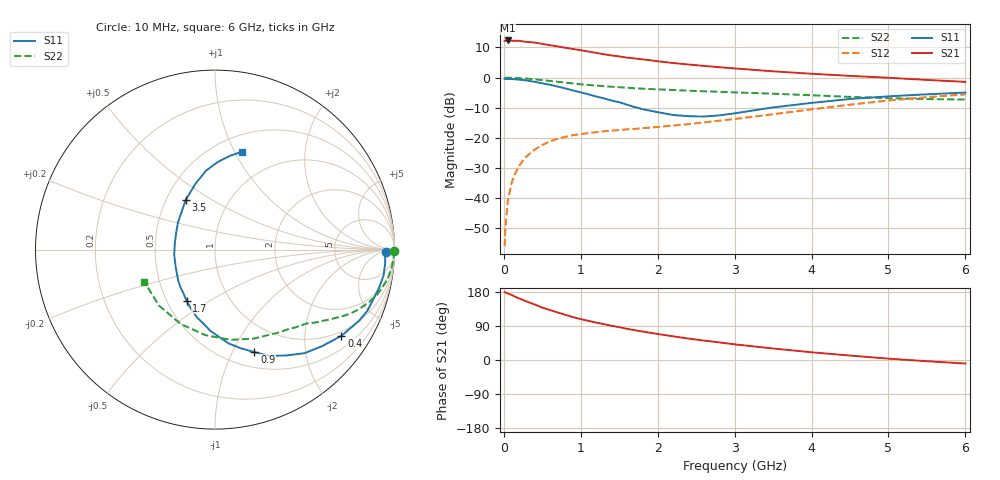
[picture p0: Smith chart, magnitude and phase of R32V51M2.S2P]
! SIEMENS Small Signal Semiconductors
! BFR181
! Si NPN RF Bipolar Junction Transistor in SOT23
! VCE = 2.5 V  IC = 1.2 mA
! Common Emitter S-Parameters:  May  1996
# GHz  S  MA  R  50
!  f  S11  S21  S12  S22
! GHz  MAG  ANG  MAG  ANG  MAG  ANG  MAG  ANG
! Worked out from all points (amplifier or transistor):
!   36 points, 10 MHz to 6 GHz, reference 50 ohm
!   highest |S21| = 12.3 dB at 50 MHz (marker M1)
!   |S21| within 3 dB of that: start of sweep to 939.8 MHz
!   unconditionally stable (mu >= 1): 1.89 GHz to 3.581 GHz
!   at 250 MHz: K = 0.17, MSG = 19.7 dB, |S12| = -27.5 dB
!   at 1.4 GHz: K = 0.82, MSG = 12.5 dB, |S12| = -17.6 dB
!   at 6 GHz: K = 0.87, MSG = 2.1 dB, |S12| = -5.6 dB
!   S11 on the Smith chart (normalised r, x): 10 MHz: 38, -12; 400 MHz: 0.86, -3.02; 900 MHz: 0.67, -1.22; 1.7 GHz: 0.63, -0.40; 3.5 GHz: 0.63, +0.39; 6 GHz: 0.67, +1.07
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0.01  0.9535 -0.9  4.077 179.4  0.0016 89.9  0.9983 -0.5
0.02  0.9489 -1.7  4.045 178.1  0.0031 87.8  0.9955 -0.9
0.05  0.9512 -4.6  4.138 175.8  0.0087 88.1  0.9968 -2.0
0.1  0.9502 -8.8  4.104 171.7  0.0178 85.7  0.9936 -4.0
0.15  0.9378 -13.2  4.086 166.5  0.0262 81.2  0.9878 -6.2
0.2  0.925 -17.4  4.08 162.4  0.0345 78.7  0.9805 -8.2
0.3  0.8956 -26.2  3.915 154.1  0.0498 73.9  0.9614 -11.9
0.4  0.8529 -34.3  3.824 146.6  0.0639 69.2  0.9386 -15.4
0.5  0.8036 -42.0  3.627 138.3  0.0763 64.5  0.9091 -18.5
0.6  0.7626 -49.2  3.449 131.9  0.0878 60.8  0.8816 -21.2
0.7  0.7101 -56.2  3.297 125.4  0.0969 57.9  0.8545 -23.6
0.9  0.6114 -69.0  2.984 113.1  0.1111 52.5  0.801 -27.6
1.1  0.5284 -81.7  2.712 103.3  0.1204 49.2  0.7561 -30.8
1.4  0.4168 -99.0  2.332 90.4  0.1317 46.5  0.7064 -34.8
1.7  0.3253 -119.2  2.085 78.7  0.141 46.4  0.6661 -37.9
1.9  0.2834 -133.1  1.945 71.9  0.1483 47.1  0.6465 -40.2
2.2  0.2401 -155.6  1.749 62.5  0.1601 48.1  0.6245 -43.9
2.8  0.2361 156.4  1.488 46.5  0.1932 51.4  0.5825 -52.4
3.5  0.3207 120.7  1.273 30.4  0.2473 51.9  0.541 -66.4
4.5  0.4426 96.5  1.069 11.7  0.3564 46.2  0.4795 -96.5
5.5  0.5292 80.9  0.916 -3.2  0.4741 33.8  0.441 -135.1
6  0.5658 74.5  0.851 -9.3  0.5271 26.0  0.433 -155.5
